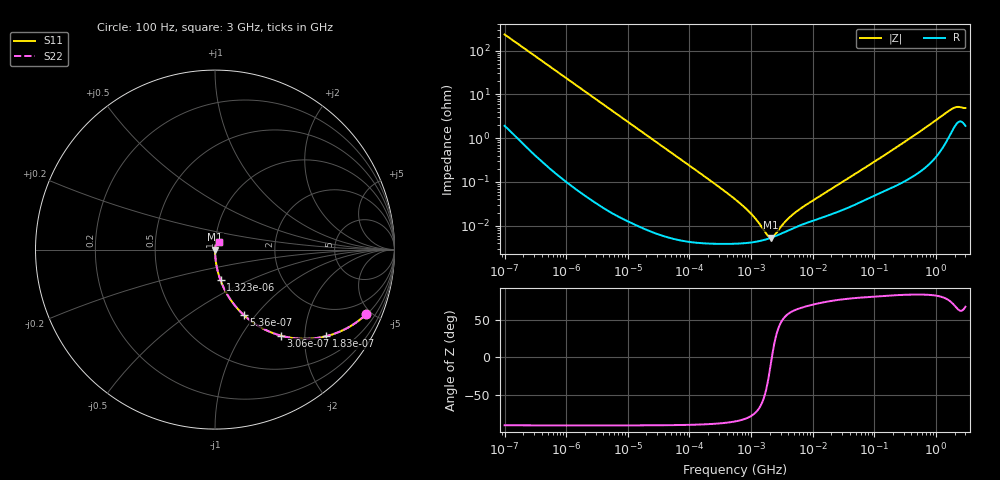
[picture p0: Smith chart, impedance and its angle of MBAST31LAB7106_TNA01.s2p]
! MBAST31LAB7106_TNA01  S-PARAMETER MODEL  ( Standard Model )
! Model Generated by TAIYO YUDEN Corporation (http://www.ty-top.com)
! Version 1.0
! TAIYO YUDEN Control No. 220601
! Copyright(c) 2012 TAIYO YUDEN CO.,LTD. All Rights Reserved.
! Product Description (link to TY-COMPAS)
! https://ds.yuden.co.jp/TYCOMPAS/or/detail?pn=MBAST31LAB7106KTNA01&u=M
! Products Name : Multilayer Ceramic Capacitors
! Characteristics :
!  Capacitance : 10 [uF] , Rated Voltage : 25 [V] , TCC : X7R
!  Case Size : 3.2 x 1.6 / 0.126 x 0.063 [mm/inch] , Thickness : 1.6 / 0.063 [mm/inch]
!  (Conditions: Temperature = 25 [degC] , DC Bias Voltage = 0 [V])
! External Node Assignments :
!  1  o---| |---o  2
! GND o---------o GND
! Frequency Range : 100Hz  -  3GHz  [ 401 STEP ]
# MHZ S RI R 50
! Freq[MHz].  S11 Real  S11 Imag  S21 Real  S21 Imag  S12 Real  S12 Imag  S22 Real  S22 Imag
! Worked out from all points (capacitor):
!   401 points, 100 Hz to 3 GHz, reference 50 ohm
!   read as one part in series: C = 6.84 uF near 109 Hz
!   lowest |Z| = 5.37 mohm at 2.08 MHz (marker M1)
!   series resonance near 2.169 MHz, so ESL is about 790 pH
!   S11 on the Smith chart (normalised r, x): 100 Hz: 1.04, -4.65; 183 Hz: 1.02, -2.55; 306 Hz: 1.01, -1.52; 536 Hz: 1.00, -0.87; 1.323 kHz: 1.00, -0.35; 3 GHz: 1.04, +0.09
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0.0001  0.8416 -0.361  0.1584 0.361  0.1584 0.361  0.8416 -0.361
0.000183  0.6186 -0.4825  0.3814 0.4825  0.3814 0.4825  0.6186 -0.4825
0.000306  0.3682 -0.4796  0.6318 0.4796  0.6318 0.4796  0.3682 -0.4796
0.000536  0.161 -0.3652  0.839 0.3652  0.839 0.3652  0.161 -0.3652
0.000789  0.0818 -0.2718  0.9182 0.2718  0.9182 0.2718  0.0818 -0.2718
0.001323  0.0311 -0.1714  0.9689 0.1714  0.9689 0.1714  0.0311 -0.1714
0.001788  0.0174 -0.1287  0.9826 0.1287  0.9826 0.1287  0.0174 -0.1287
0.005476  0.00203 -0.0428  0.998 0.0428  0.998 0.0428  0.00203 -0.0428
0.031977  0.000117 -0.00738  0.9999 0.00738  0.9999 0.00738  0.000117 -0.00738
0.547723  3.91e-05 -0.000403  1 0.000403  1 0.000403  3.91e-05 -0.000403
0.918067  4.1e-05 -0.000209  1 0.000209  1 0.000209  4.1e-05 -0.000209
1.411895  4.53e-05 -9.41e-05  1 9.41e-05  1 9.41e-05  4.53e-05 -9.41e-05
1.6065  4.74e-05 -6.43e-05  1 6.43e-05  1 6.43e-05  4.74e-05 -6.43e-05
2.079876  5.3e-05 -8.64e-06  0.9999 8.64e-06  0.9999 8.64e-06  5.3e-05 -8.64e-06
2.81117  6.27e-05 5.25e-05  0.9999 -5.25e-05  0.9999 -5.25e-05  6.27e-05 5.25e-05
3.198641  6.79e-05 7.83e-05  0.9999 -7.83e-05  0.9999 -7.83e-05  6.79e-05 7.83e-05
5.135543  9.14e-05 0.000176  0.9999 -0.000176  0.9999 -0.000176  9.14e-05 0.000176
9.794414  0.000129 0.000346  0.9999 -0.000346  0.9999 -0.000346  0.000129 0.000346
175.1444  0.000716 0.00477  0.9993 -0.00477  0.9993 -0.00477  0.000716 0.00477
1789.813  0.0154 0.0427  0.9846 -0.0427  0.9846 -0.0427  0.0154 0.0427
2219.584  0.0238 0.0446  0.9762 -0.0446  0.9762 -0.0446  0.0238 0.0446
3000  0.0206 0.0431  0.9794 -0.0431  0.9794 -0.0431  0.0206 0.0431
